FUNCTION "FC_TRASLAZ_KLASKA" : VOID
TITLE =CENTRATORE 1
VERSION : 0.1


VAR_TEMP
  App_Pos_Attuale : REAL ;
  Pos_Toll_Max : REAL ;
  Pos_Toll_Min : REAL ;
  App_Pos_Impostata : REAL ;
END_VAR
BEGIN
NETWORK
TITLE =LETTURA STATUS WORD DA DRIVE
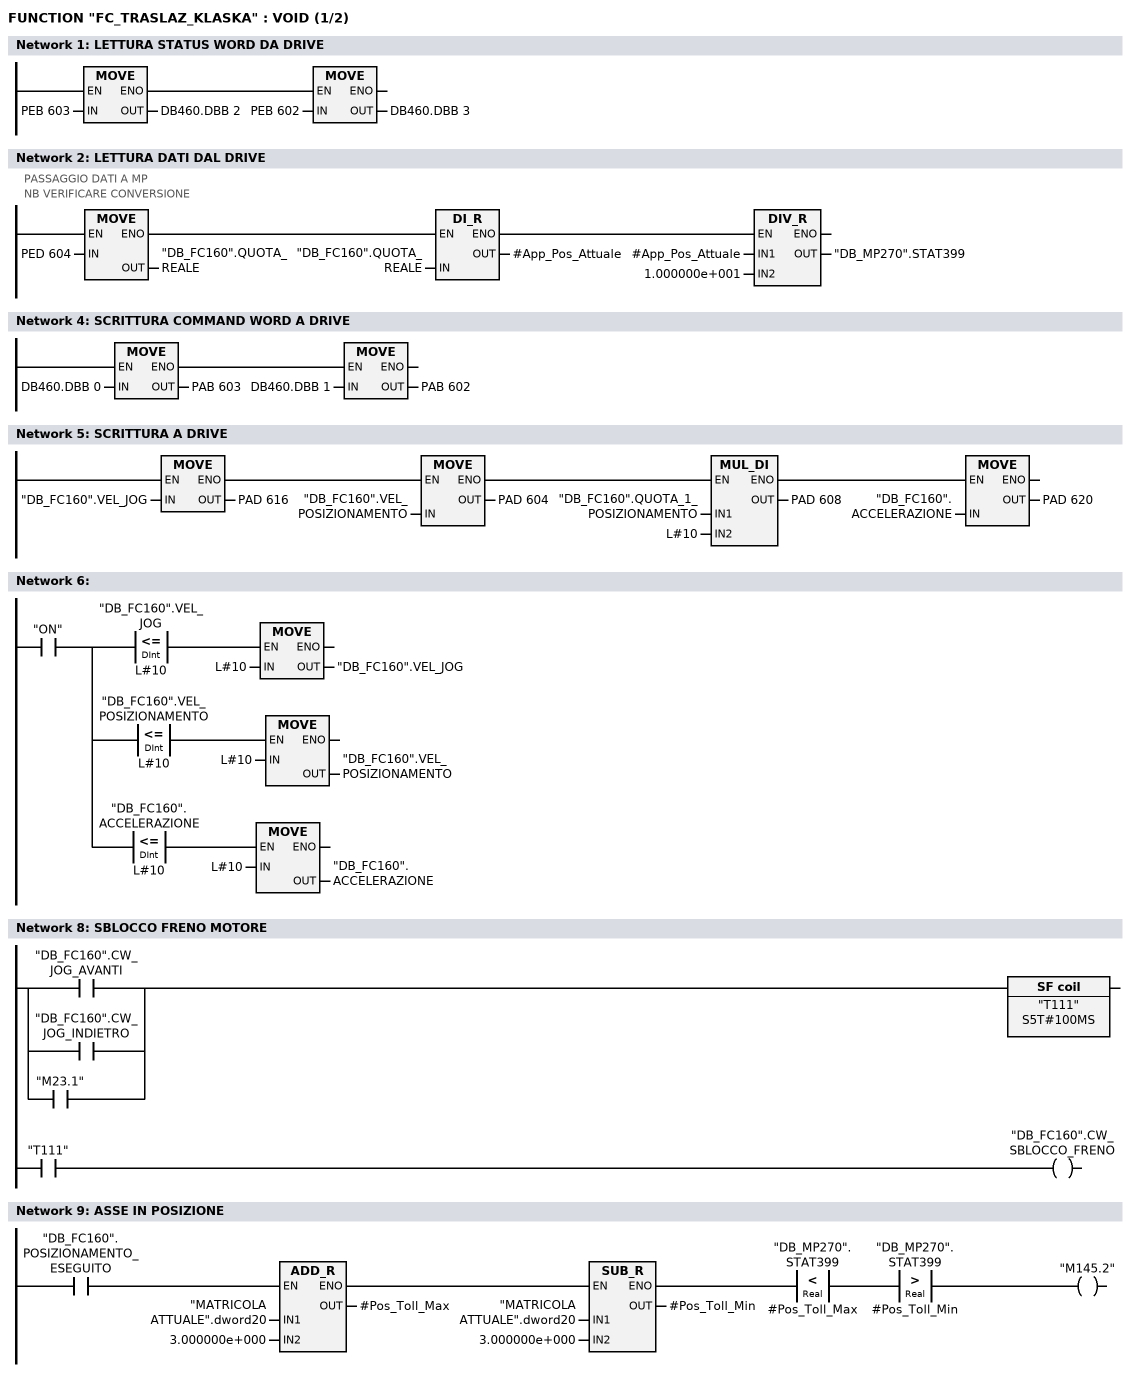
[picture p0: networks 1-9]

      U(    ;
      L     PEB  603;
      T     DB460.DBB    2;
      SET   ;
      SAVE  ;
      CLR   ;
      U     BIE;
      )     ;
      SPBNB _001;
      L     PEB  602;
      T     DB460.DBB    3;
_001: NOP   0;
NETWORK
TITLE =LETTURA DATI DAL DRIVE
//PASSAGGIO DATI A MP
//
//NB VERIFICARE CONVERSIONE
      U(    ;
      U(    ;
      L     PED  604;
      T     "DB_FC160".QUOTA_REALE;
      SET   ;
      SAVE  ;
      CLR   ;
      U     BIE;
      )     ;
      SPBNB _002;
      L     "DB_FC160".QUOTA_REALE;
      DTR   ;
      T     #App_Pos_Attuale;
      SET   ;
      SAVE  ;
      CLR   ;
_002: U     BIE;
      )     ;
      SPBNB _003;
      L     #App_Pos_Attuale;
      L     1.000000e+001;
      /R    ;
      T     "DB_MP270".STAT399;
_003: NOP   0;
NETWORK
TITLE =

NETWORK
TITLE =SCRITTURA COMMAND WORD A DRIVE

      U(    ;
      L     DB460.DBB    0;
      T     PAB  603;
      SET   ;
      SAVE  ;
      CLR   ;
      U     BIE;
      )     ;
      SPBNB _004;
      L     DB460.DBB    1;
      T     PAB  602;
_004: NOP   0;
NETWORK
TITLE =SCRITTURA A DRIVE

      U(    ;
      U(    ;
      U(    ;
      L     "DB_FC160".VEL_JOG;
      T     PAD  616;
      SET   ;
      SAVE  ;
      CLR   ;
      U     BIE;
      )     ;
      SPBNB _005;
      L     "DB_FC160".VEL_POSIZIONAMENTO;
      T     PAD  604;
      SET   ;
      SAVE  ;
      CLR   ;
_005: U     BIE;
      )     ;
      SPBNB _006;
      L     "DB_FC160".QUOTA_1_POSIZIONAMENTO;
      L     L#10;
      *D    ;
      T     PAD  608;
      UN    OV;
      SAVE  ;
      CLR   ;
_006: U     BIE;
      )     ;
      SPBNB _007;
      L     "DB_FC160".ACCELERAZIONE;
      T     PAD  620;
_007: NOP   0;
NETWORK
TITLE =

      U     "ON";
      =     L     16.0;
      U     L     16.0;
      U(    ;
      L     "DB_FC160".VEL_JOG;
      L     L#10;
      <=D   ;
      )     ;
      SPBNB _008;
      L     L#10;
      T     "DB_FC160".VEL_JOG;
_008: NOP   0;
      U     L     16.0;
      U(    ;
      L     "DB_FC160".VEL_POSIZIONAMENTO;
      L     L#10;
      <=D   ;
      )     ;
      SPBNB _009;
      L     L#10;
      T     "DB_FC160".VEL_POSIZIONAMENTO;
_009: NOP   0;
      U     L     16.0;
      U(    ;
      L     "DB_FC160".ACCELERAZIONE;
      L     L#10;
      <=D   ;
      )     ;
      SPBNB _00a;
      L     L#10;
      T     "DB_FC160".ACCELERAZIONE;
_00a: NOP   0;
NETWORK
TITLE =

NETWORK
TITLE =SBLOCCO FRENO MOTORE

      U(    ;
      O     "DB_FC160".CW_JOG_AVANTI;
      O     "DB_FC160".CW_JOG_INDIETRO;
      O     "M23.1";
      )     ;
      L     S5T#100MS;
      SA    "T111";
      NOP   0;
      NOP   0;
      NOP   0;
      U     "T111";
      =     "DB_FC160".CW_SBLOCCO_FRENO;
NETWORK
TITLE =ASSE IN POSIZIONE

      U(    ;
      U(    ;
      U     "DB_FC160".POSIZIONAMENTO_ESEGUITO;
      SPBNB _00b;
      L     "MATRICOLA ATTUALE".dword20;
      L     3.000000e+000;
      +R    ;
      T     #Pos_Toll_Max;
      UN    OV;
      SAVE  ;
      CLR   ;
_00b: U     BIE;
      )     ;
      SPBNB _00c;
      L     "MATRICOLA ATTUALE".dword20;
      L     3.000000e+000;
      -R    ;
      T     #Pos_Toll_Min;
      UN    OV;
      SAVE  ;
      CLR   ;
_00c: U     BIE;
      )     ;
      U(    ;
      L     "DB_MP270".STAT399;
      L     #Pos_Toll_Max;
      <R    ;
      )     ;
      U(    ;
      L     "DB_MP270".STAT399;
      L     #Pos_Toll_Min;
      >R    ;
      )     ;
      =     "M145.2";
NETWORK
TITLE =START POSIZIONAMENTO ASSE KLASCKA
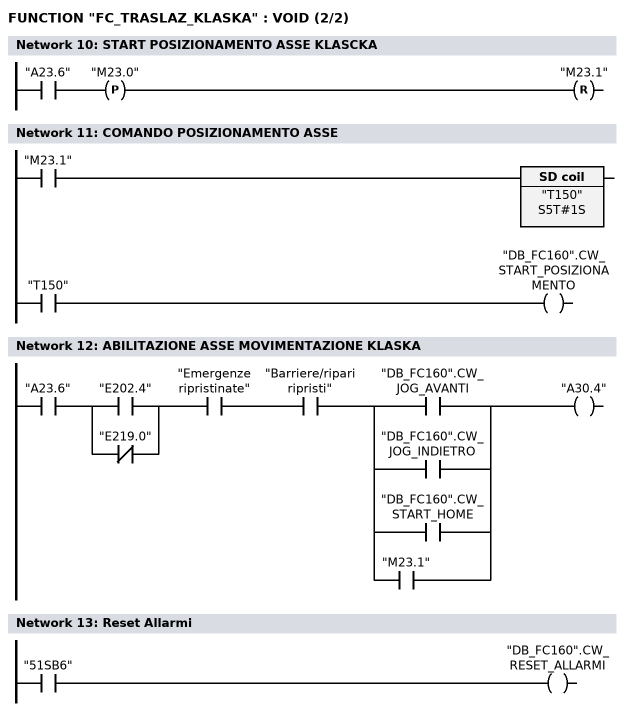
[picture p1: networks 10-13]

      U     "A23.6";
      FP    "M23.0";
      R     "M23.1";
NETWORK
TITLE =COMANDO POSIZIONAMENTO ASSE

      U     "M23.1";
      L     S5T#1S;
      SE    "T150";
      NOP   0;
      NOP   0;
      NOP   0;
      U     "T150";
      =     "DB_FC160".CW_START_POSIZIONAMENTO;
NETWORK
TITLE =ABILITAZIONE ASSE MOVIMENTAZIONE KLASKA

      U     "A23.6";
      U(    ;
      O     "E202.4";
      ON    "E219.0";
      )     ;
      U     "Emergenze ripristinate";
      U     "Barriere/ripari ripristi";
      U(    ;
      O     "DB_FC160".CW_JOG_AVANTI;
      O     "DB_FC160".CW_JOG_INDIETRO;
      O     "DB_FC160".CW_START_HOME;
      O     "M23.1";
      )     ;
      =     "A30.4";
NETWORK
TITLE =Reset Allarmi

      U     "51SB6";
      =     "DB_FC160".CW_RESET_ALLARMI;
NETWORK
TITLE =Posizione Impostata

      U     "ON";
      =     L     16.0;
      U     L     16.0;
      U     "Modo man.";
      UN    "Cambio produz. in corso";
      =     L     16.1;
      U     L     16.1;
      U     "M144.0";
      FP    "M145.0";
      SPBNB _00d;
      L     "MATRICOLA ATTUALE".dword20;
      L     1.000000e+001;
      +R    ;
      T     "MATRICOLA ATTUALE".dword20;
_00d: NOP   0;
      U     L     16.1;
      U     "M144.1";
      FP    "M145.1";
      SPBNB _00e;
      L     "MATRICOLA ATTUALE".dword20;
      L     1.000000e+001;
      -R    ;
      T     "MATRICOLA ATTUALE".dword20;
_00e: NOP   0;
      U     L     16.0;
      U(    ;
      L     "MATRICOLA ATTUALE".dword20;
      L     0.000000e+000;
      <R    ;
      )     ;
      SPBNB _00f;
      L     0.000000e+000;
      T     "MATRICOLA ATTUALE".dword20;
_00f: NOP   0;
      U     L     16.0;
      U(    ;
      L     "MATRICOLA ATTUALE".dword20;
      L     7.000000e+002;
      >R    ;
      )     ;
      SPBNB _010;
      L     7.000000e+002;
      T     "MATRICOLA ATTUALE".dword20;
_010: NOP   0;
      U(    ;
      U     L     16.0;
      SPBNB _011;
      L     "MATRICOLA ATTUALE".dword20;
      L     1.000000e+000;
      *R    ;
      T     #App_Pos_Impostata;
      UN    OV;
      SAVE  ;
      CLR   ;
_011: U     BIE;
      )     ;
      SPBNB _012;
      L     #App_Pos_Impostata;
      RND-  ;
      T     "DB_FC160".QUOTA_1_POSIZIONAMENTO;
_012: NOP   0;
NETWORK
TITLE =

NETWORK
TITLE =AZZERAMENTO ENCODER ASSOLUTO
//L'AZZERAMENTO VIENE ESEGUITO SOLO CON IL MOTORE ABILITATO
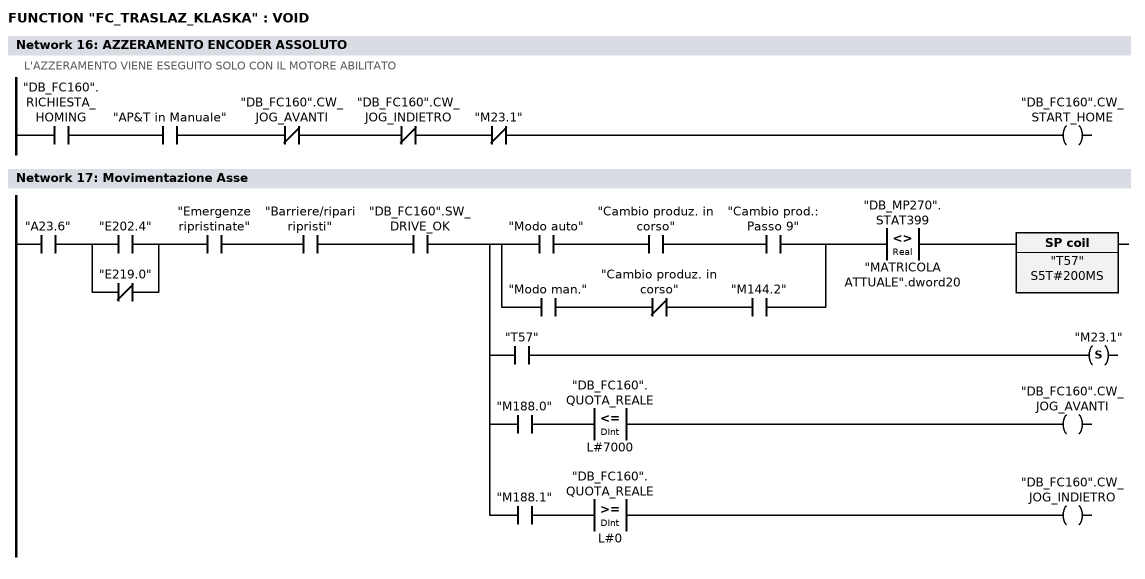
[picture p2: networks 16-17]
      U     "DB_FC160".RICHIESTA_HOMING;
      U     "AP&T in Manuale";
      UN    "DB_FC160".CW_JOG_AVANTI;
      UN    "DB_FC160".CW_JOG_INDIETRO;
      UN    "M23.1";
      =     "DB_FC160".CW_START_HOME;
NETWORK
TITLE =Movimentazione Asse

      U     "A23.6";
      U(    ;
      O     "E202.4";
      ON    "E219.0";
      )     ;
      U     "Emergenze ripristinate";
      U     "Barriere/ripari ripristi";
      U     "DB_FC160".SW_DRIVE_OK;
      =     L     16.0;
      U     L     16.0;
      U(    ;
      U     "Modo auto";
      U     "Cambio produz. in corso";
      U     "Cambio prod.: Passo 9";
      O     ;
      U     "Modo man.";
      UN    "Cambio produz. in corso";
      U     "M144.2";
      )     ;
      U(    ;
      L     "DB_MP270".STAT399;
      L     "MATRICOLA ATTUALE".dword20;
      <>R   ;
      )     ;
      L     S5T#200MS;
      SI    "T57";
      NOP   0;
      NOP   0;
      NOP   0;
      NOP   0;
      U     L     16.0;
      U     "T57";
      S     "M23.1";
      U     L     16.0;
      U     "M188.0";
      U(    ;
      L     "DB_FC160".QUOTA_REALE;
      L     L#7000;
      <=D   ;
      )     ;
      =     "DB_FC160".CW_JOG_AVANTI;
      U     L     16.0;
      U     "M188.1";
      U(    ;
      L     "DB_FC160".QUOTA_REALE;
      L     L#0;
      >=D   ;
      )     ;
      =     "DB_FC160".CW_JOG_INDIETRO;
NETWORK
TITLE =

      U     "ON";
      =     L     16.0;
      U     L     16.0;
      U     "M23.1";
      =     L     16.1;
      U     L     16.1;
      FP    "DB_FC160".FP_1;
      S     "DB_FC160".APPOGGIO_1;
      R     "DB_FC160".POSIZIONAMENTO_ESEGUITO;
      U(    ;
      U     L     16.1;
      U     "DB_FC160".APPOGGIO_1;
      L     S5T#1S;
      SE    T    170;
      NOP   0;
      NOP   0;
      NOP   0;
      U     T    170;
      )     ;
      FP    "DB_FC160".FP_11;
      S     "DB_FC160".APPOGGIO_2;
      U     L     16.1;
      U     "DB_FC160".APPOGGIO_2;
      U     "DB_FC160".SW_POSIZ_ESEGUITO;
      S     "DB_FC160".POSIZIONAMENTO_ESEGUITO;
      R     "M23.1";
      U     L     16.0;
      UN    "M23.1";
      R     "DB_FC160".APPOGGIO_1;
      R     "DB_FC160".APPOGGIO_2;
      U     L     16.0;
      U     "OFF";
      R     "DB_FC160".POSIZIONAMENTO_ESEGUITO;
END_FUNCTION

